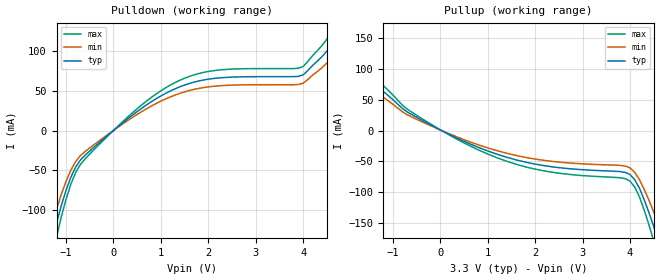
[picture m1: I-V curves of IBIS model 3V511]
[IBIS Ver]   2.1
[File name]   671-01_3.ibs
[File Rev]   2.0
[Date]   08/21/00
[Source]   ICS MicroClock Applications Engineering 2
[Disclaimer] This information is for modeling purposes only, and is
(C) Copyright Integrated Circuit Systems, Inc. 1997-2001
   All rights reserved
ICS hereby grants the user of this IBIS model a non-exclusive,
nontransferable license to use this IBIS model under the following terms.
Before using this IBIS model, the user should read this license.
If the user does not accept these terms,  the IBIS model should be
returned to ICS within 30 days.
   The user is granted this license only to use the IBIS model and
is not granted rights to sell, load, rent, lease or license the IBIS
model in whole or in part, or in modified form to anyone other than
user. User may modify the IBIS model to suit its specific
applications but rights to derivative works and such modifications
shall belong to ICS.
   This IBIS model is provided on an "AS IS" basis and ICS makes
absolutely no warranty with respect to the information contained
herein. ICS DISCLAIMS AND CUSTOMER WAIVES ALL WARRANTIES, EXPRESS
OR IMPLIED, INCLUDING WARRANTIES OF MERCHANTABILITY OR FITNESS FOR
A PARTICULAR PURPOSE. The entire risk as to quality and performance
is with the Customer. ACCORDINGLY, IN NO EVENT SHALL THE COMPANY BE
LIABLE FOR ANY DAMAGES, WHETHER IN CONTRACT OR TORT,INCLUDING ANY
LOST PROFITS OR OTHER INCIDENTAL, CONSEQUENTIAL, EXEMPLARY, OR
PUNITIVE DAMAGES ARISING OUT OF THE USE OR APPLICATION OF THE IBIS
model provided in this package. Further, ICS reserves the right to
make changes without notice to any product herein to improve
reliability, function, or design. ICS does not convey any license
under patent rights or any other intellectual property rights,
including those of third parties.
   ICS is not obligated to provide maintenance or support
for the licensed IBIS model.
[Component]   ICS671-01
[Manufacturer] Integrated Circuit Systems Inc.
[Package]
|   typ   min   max
R_pkg   40m   35m   45m
L_pkg   1.65nH   1.35nH   1.95nH
C_pkg   0.24pF   0.14pF   0.34pF
[pin]   signal_name   model_name   R_pin   L_pin   C_pin
   2   CLK1   3V511
   3   CLK2   3V511
   6   CLK3   3V511
   7   CLK4   3V511
   10   CLK5   3V511
   11   CLK6   3V511
   14   CLK7   3V511
   15   CLK8   3V511
| Models and submodels in the file (1): 3V511 (Output)
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|   ICS671-01 3.3V Clock Drive Model
| This model is suitable for all output pins on the
| ICS671-01
[Model]   3V511
Model_type   Output
Polarity   Non-Inverting
|   typ   min   max
C_comp   5pF   4pF   6pF
|   typ   min   max
[Voltage range]  3.3V   2.94V   3.63V
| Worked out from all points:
|   slope of the pulldown table from 0 to 0.495 V, typ, clamps not added: 21.1 ohm
|   slope of the pullup table from 0 to 0.495 V, typ, clamps not added: 27 ohm
[pulldown]
|Voltage I (typ)   I (min)   I (max)
-3.3V     -3A        -3A        -3A
-1.4V     -163.3mA   -138.9mA   -187.8mA
-1.2V     -116.3mA   -98.86mA   -133.8mA
-900mV    -58.78mA   -49.96mA   -67.59mA
-700mV    -37.16mA   -31.59mA   -42.73mA
500mV     23.74mA    20.18mA    27.3mA
1.4V      54.72mA    46.51mA    62.93mA
4V        69.71mA    59.26mA    80.17mA
4.5V      99.55mA    84.62mA    114.5mA
4.7V      124.4mA    105.7mA    143mA
4.9V      166.7mA    141.7mA    191.7mA
6.6V      3A         3A         3A
[pullup]
|Voltage I (typ)   I (min)   I (max)
-3.3V     3A         3A         3A
-2.2V     178.3mA    151.5mA    205mA
-2.1V     158.9mA    135mA      182.7mA
-1.8V     109.5mA    93.05mA    125.9mA
-1.4V     76.99mA    65.45mA    88.54mA
-700mV    30.37mA    25.82mA    34.93mA
200mV     -6.72mA    -5.71mA    -7.73mA
1.8V      -51.44mA   -43.72mA   -59.15mA
4V        -71.53mA   -60.8mA    -82.26mA
4.5V      -156.2mA   -132.8mA   -179.6mA
4.7V      -199.9mA   -169.9mA   -229.9mA
6.6V      -3A        -3A        -3A
[Ramp]
|   typ   min   max
dV/dt_r   1.31/0.41n   1.24/0.45n   1.37/0.37n
dV/dt_f   1.54/0.34n   1.46/0.38n   1.62/0.31n
